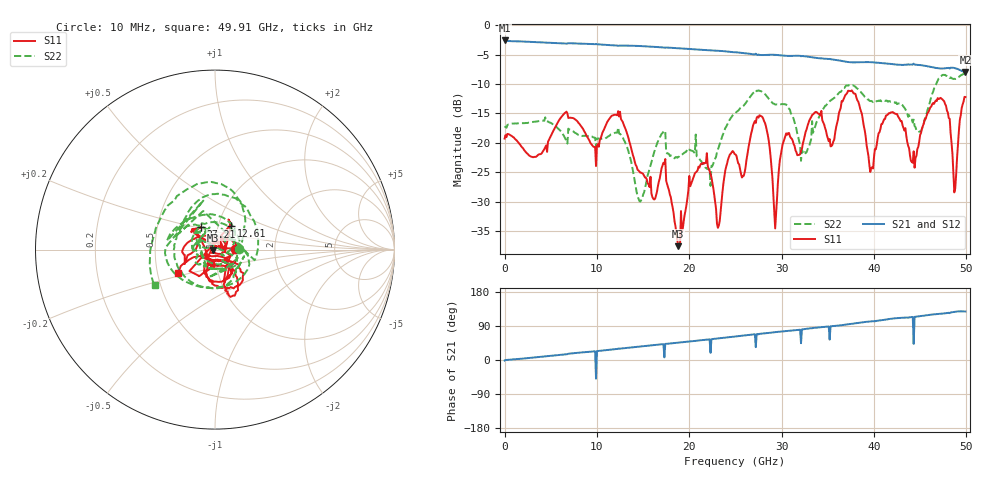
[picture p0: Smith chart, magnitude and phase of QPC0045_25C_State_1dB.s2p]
!File name = QPC0045_25C_State_1dB.s2p
!Date Time: 2024/05/02 05:42:16 AM
!Cal Ref Plane:TRL
!TEMP = 25C
!Vdd(V) = 3.15
!Vss(V) = 0.000
# GHz  S  DB  R  50
!%	Freq(GHz)  S11(dB)  S11(deg)  S21(dB)  S21(deg)  S12(dB)  S12(deg)  S22(dB)  S22(deg)
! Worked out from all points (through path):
!   500 points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, 10 MHz to 49.91 GHz, reference 50 ohm
!   highest |S21| = -2.60 dB at 10 MHz (marker M1); lowest = -8.0 dB at 49.91 GHz (marker M2)
!   lowest |S11| = -37.6 dB at 18.81 GHz (marker M3), VSWR 1.03, Z = 48.7 - j0.341 ohm
!   |S11| at or under -10 dB: start of sweep to end of sweep
!   |S22| runs from -30.0 to -8.2 dB; largest |S21 - S12| = 0.0023
!   S11 on the Smith chart (normalised r, x): 10 MHz: 1.24, +0.00; 12.61 GHz: 1.15, +0.31; 27.21 GHz: 0.83, +0.21; 49.91 GHz: 0.64, -0.18
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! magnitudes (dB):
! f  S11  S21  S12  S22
! 10 MHz  -19.3  -2.6  -2.6  -17.4
! 8.41 GHz  -17.4  -3.1  -3.1  -18.8
! 12.61 GHz  -16.0  -3.5  -3.5  -18.6
! 14.71 GHz  -25.1  -3.6  -3.5  -30.0
! 16.71 GHz  -26.6  -3.7  -3.7  -19.4
! 18.81 GHz  -37.6  -3.9  -3.9  -22.4
! 21.11 GHz  -24.2  -4.2  -4.2  -22.7
! 23.21 GHz  -34.0  -4.4  -4.3  -20.7
! 25.01 GHz  -22.0  -4.6  -4.6  -14.9
! 27.21 GHz  -16.6  -4.8  -4.8  -11.0
! 28.41 GHz  -17.9  -5.0  -5.0  -12.1
! 29.31 GHz  -34.5  -5.0  -5.0  -13.5
! 30.31 GHz  -19.3  -5.2  -5.2  -13.4
! 33.31 GHz  -15.3  -5.4  -5.4  -16.3
! 35.51 GHz  -20.3  -5.8  -5.8  -12.6
! 37.81 GHz  -11.6  -6.3  -6.3  -10.3
! 39.71 GHz  -24.3  -6.3  -6.3  -12.9
! 41.61 GHz  -15.0  -6.5  -6.5  -12.9
! 44.21 GHz  -23.4  -6.7  -6.7  -16.5
! 47.41 GHz  -12.6  -7.4  -7.4  -8.5
! 48.81 GHz  -27.7  -7.3  -7.3  -9.2
! 49.91 GHz  -12.2  -8.0  -8.0  -8.3
